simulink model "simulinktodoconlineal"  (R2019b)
settings: Solver=VariableStepAuto  StartTime=0.0  StopTime=90  RelTol=1e-3
libraries: cstblocks x6

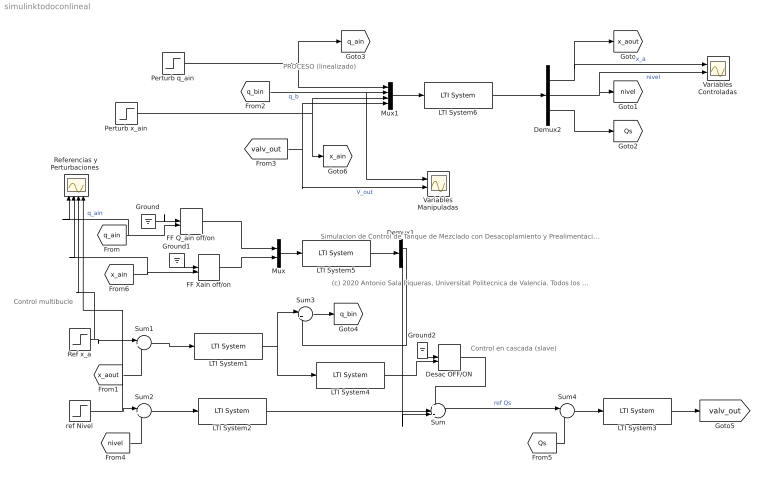
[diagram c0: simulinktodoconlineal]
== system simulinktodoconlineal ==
  note: (c) 2020 Antonio Sala Piqueras, Universitat Politecnica de Valencia. Todos los derechos reservados
  note: Simulacion de Control de Tanque de Mezclado con Desacoplamiento y Prealimentacion (modelo lineal )
  note: PROCESO (linealizado)
  note: Control multibucle
  note: Control en cascada (slave)
  Demux1 : Demux  Outputs=2
  Demux2 : Demux  Outputs=3
  Desac OFF/ON : ManualSwitch  CurrentSetting=0
  FF Q_ain off/on : ManualSwitch  CurrentSetting=0
  FF Xain off/on : ManualSwitch  CurrentSetting=0
  Ground : Ground
  Ground1 : Ground
  Ground2 : Ground
  LTI System1 : cstblocks/LTI System  sys=K_conc  IC=[]
  LTI System2 : cstblocks/LTI System  sys=K_nivel  IC=[]
  LTI System3 : cstblocks/LTI System  sys=K_caudal  IC=[]
  LTI System4 : cstblocks/LTI System  sys=DesacQbToQs  IC=[]
  LTI System5 : cstblocks/LTI System  sys=FF_tf  IC=[]
  LTI System6 : cstblocks/LTI System  sys=G  IC=[]
  Mux : Mux  Inputs=2
  Mux1 : Mux
  Perturb q_ain : Step  Time=50  SampleTime=0
  Perturb x_ain : Step  Time=70  After=.1  SampleTime=0
  Ref x_a : Step  Time=10  After=.1  SampleTime=0
  "Referencias y Perturbaciones " : Scope  NumInputPorts=4
  Sum : Sum  Inputs=+++
  Sum1 : Sum  Inputs=|+-
  Sum2 : Sum  Inputs=|+-
  Sum3 : Sum  Inputs=|++
  Sum4 : Sum  Inputs=|+-
  Variables Controladas : Scope  NumInputPorts=2
  Variables Manipuladas : Scope  NumInputPorts=2
  ref Nivel : Step  Time=30  SampleTime=0
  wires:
  Sum/1 -> Sum4/1  "ref Qs"
  LTI System3/1 -> [valv_out]
  LTI System1/1 -> LTI System4/1, Sum3/1
  Ref x_a/1 -> Sum1/1, "Referencias y Perturbaciones "/3
  ref Nivel/1 -> Sum2/1, "Referencias y Perturbaciones "/4
  Sum2/1 -> LTI System2/1
  Sum1/1 -> LTI System1/1
  Sum3/1 -> [q_bin]
  Demux1/1 -> Sum3/2
  Demux1/2 -> Sum/3
  Mux1/1 -> LTI System6/1
  LTI System6/1 -> Demux2/1
  Demux2/1 -> Variables Controladas/1, [x_aout]  "x_a"
  Demux2/2 -> Variables Controladas/2, [nivel]  "nivel"
  Demux2/3 -> [Qs]
  Perturb q_ain/1 -> [q_ain], Mux1/1
  [q_bin] -> Variables Manipuladas/1, Mux1/2  "q_b"
  Perturb x_ain/1 -> [x_ain], Mux1/3
  [valv_out] -> Variables Manipuladas/2, Mux1/4  "V_out"
  [x_aout] -> Sum1/2
  [nivel] -> Sum2/2
  Sum4/1 -> LTI System3/1
  [Qs] -> Sum4/2
  LTI System2/1 -> Sum/2
  Mux/1 -> LTI System5/1
  LTI System5/1 -> Demux1/1
  Desac OFF/ON/1 -> Sum/1
  LTI System4/1 -> Desac OFF/ON/2
  FF Xain off/on/1 -> Mux/2
  [x_ain] -> FF Xain off/on/2, "Referencias y Perturbaciones "/2
  FF Q_ain off/on/1 -> Mux/1
  [q_ain] -> FF Q_ain off/on/2, "Referencias y Perturbaciones "/1  "q_ain"
  Ground/1 -> FF Q_ain off/on/1
  Ground1/1 -> FF Xain off/on/1
  Ground2/1 -> Desac OFF/ON/1
